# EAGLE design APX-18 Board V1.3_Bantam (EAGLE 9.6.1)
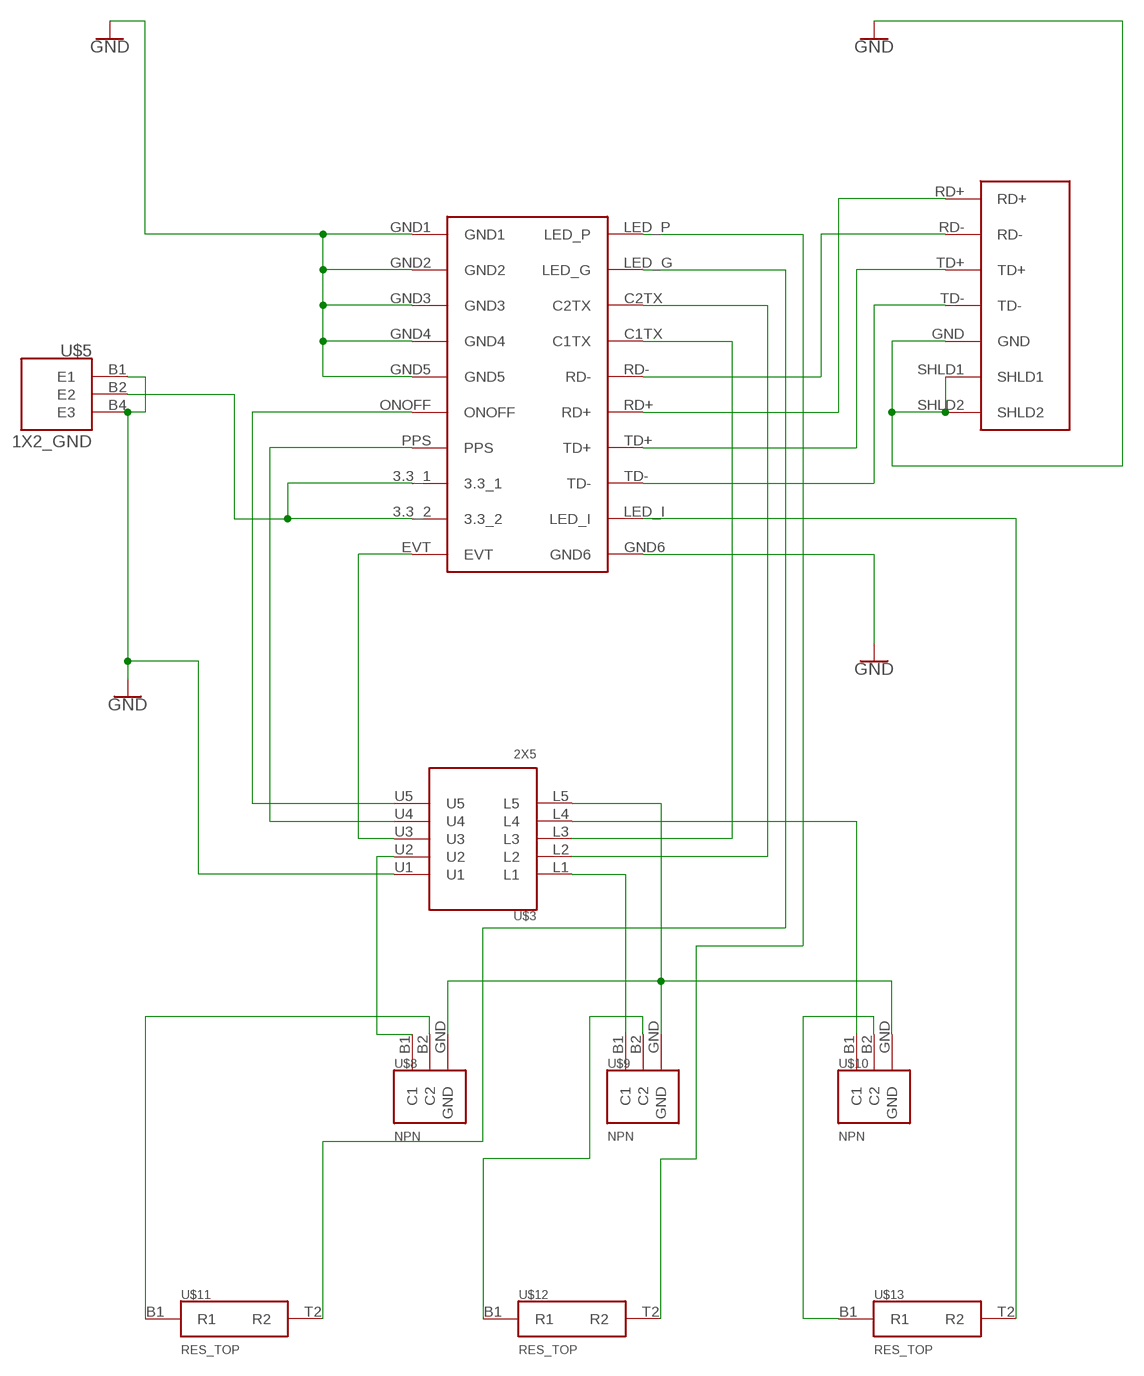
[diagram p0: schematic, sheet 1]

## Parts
U$1  APX18  [F_APX18]
U$2  MOLEX_MAG_ETH  [F_MOLEX_MAG_ETH]
U$3  2X5  [F_2X5]
U$5  1X2_GND  [F_1X2_GND]
U$8  NPN  [F_NPN]
U$9  NPN  [F_NPN]
U$10  NPN  [F_NPN]
U$11  RES_TOP  [F_RES]
U$12  RES_TOP  [F_RES]
U$13  RES_TOP  [F_RES]

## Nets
GND: U$1.GND1 U$1.GND2 U$1.GND3 U$1.GND4 U$1.GND5 U$1.GND6 U$2.GND U$2.SHLD1 U$2.SHLD2 U$3.U1 U$5.B1(E1) U$5.B4(E3)
N$1: U$1.TD- U$2.TD-
N$2: U$1.TD+ U$2.TD+
N$3: U$1.RD+ U$2.RD+
N$4: U$1.RD- U$2.RD-
N$5: U$1.3.3_1 U$1.3.3_2 U$5.B2(E2)
N$6: U$1.EVT U$3.U3
N$7: U$3.U2 U$8.B1(C1)
N$8: U$1.PPS U$3.U4
N$9: U$1.ONOFF U$3.U5
N$10: U$1.LED_I U$13.T2(R2)
N$11: U$1.C1TX U$3.L3
N$12: U$8.B2(C2) U$11.B1(R1)
N$13: U$1.C2TX U$3.L2
N$14: U$1.LED_G U$11.T2(R2)
N$15: U$1.LED_P U$12.T2(R2)
N$16: U$3.L1 U$9.B1(C1)
N$17: U$9.B2(C2) U$12.B1(R1)
N$18: U$3.L4 U$10.B1(C1)
N$19: U$10.B2(C2) U$13.B1(R1)
N$20: U$3.L5 U$8.GND U$9.GND U$10.GND

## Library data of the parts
U$1 = OpenMMS_Bantam:APX18
U$2 = OpenMMS_Bantam:MOLEX_MAG_ETH
U$3 = OpenMMS_Bantam:2X5
U$5 = OpenMMS_Bantam:1X2_GND
U$8-U$10 = OpenMMS_Bantam:NPN
U$11-U$13 = OpenMMS_Bantam:RES_TOP

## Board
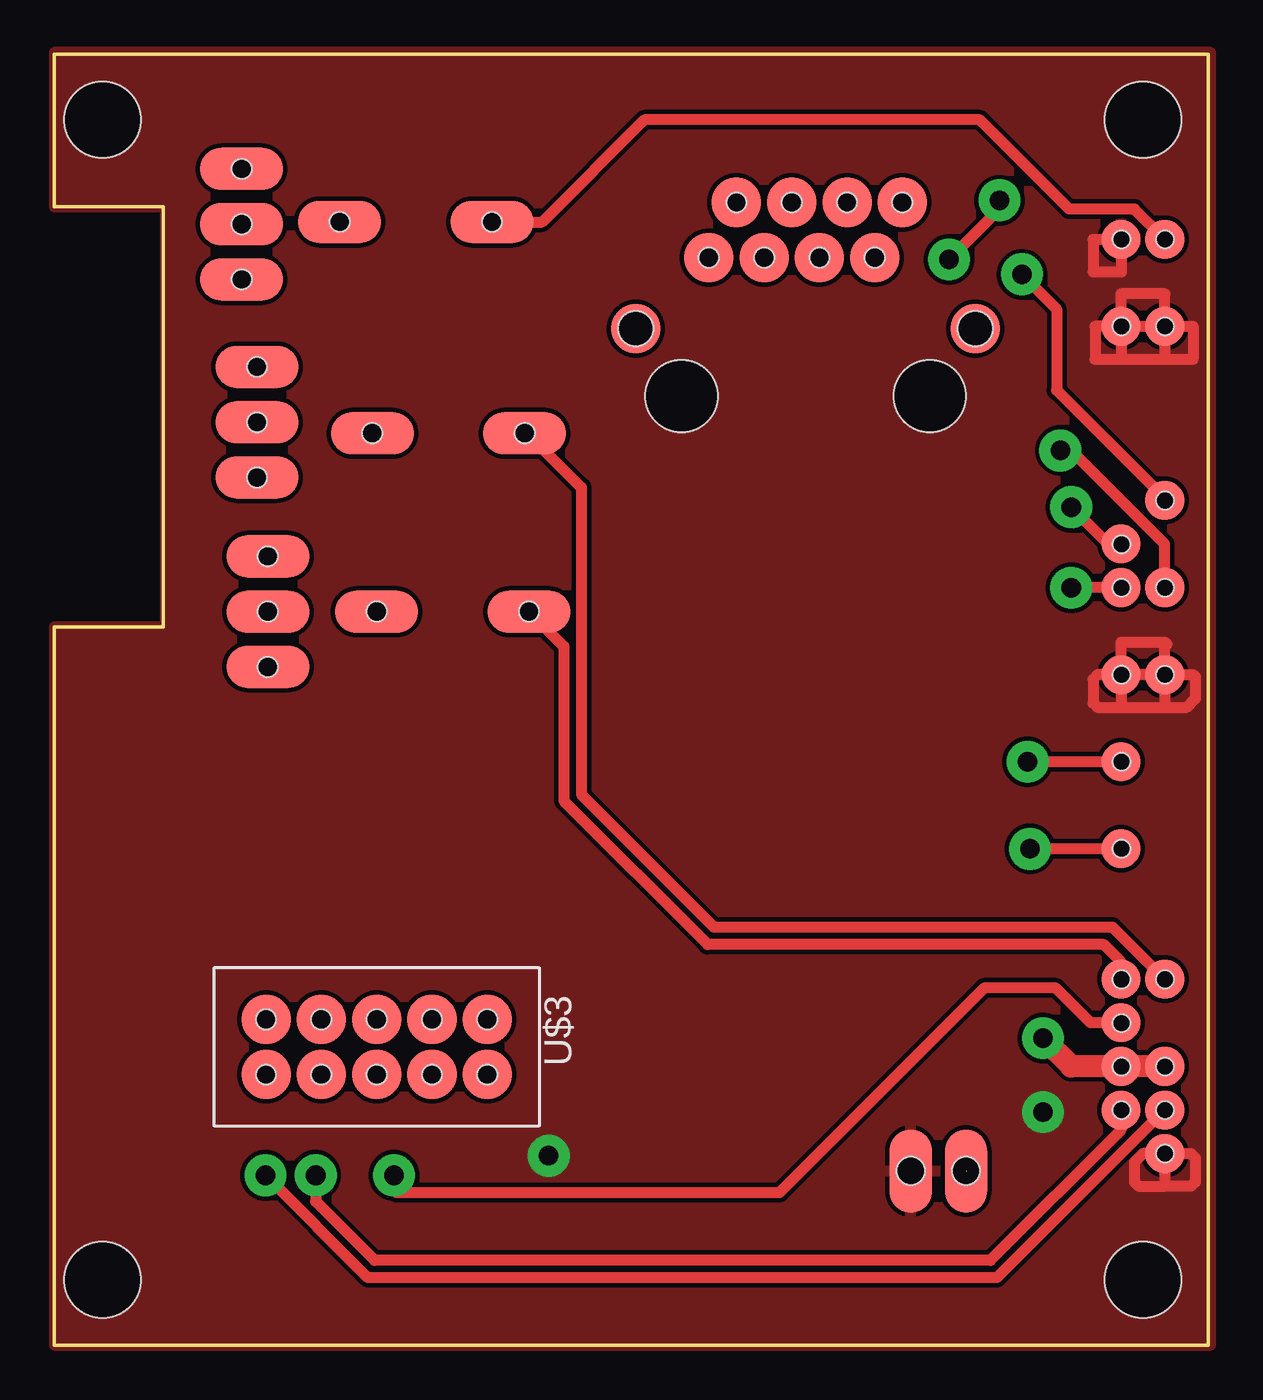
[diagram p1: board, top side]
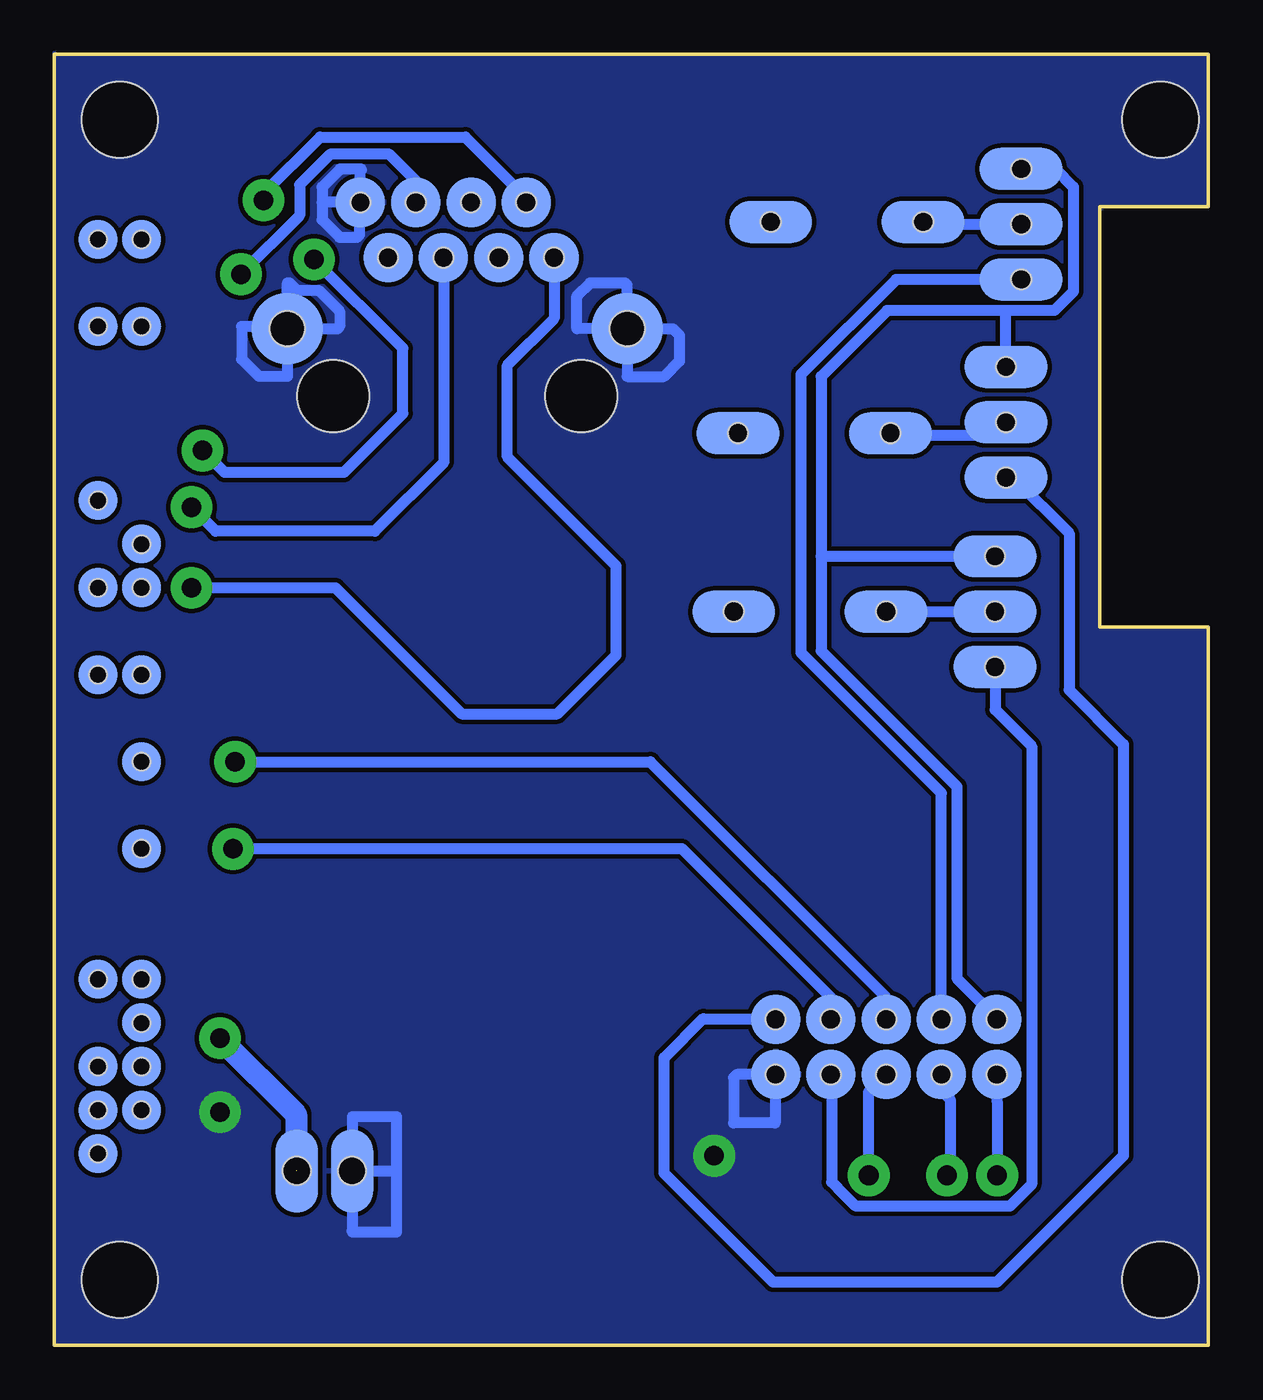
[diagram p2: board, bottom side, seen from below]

Size 53 x 59.3 mm. Coordinates in mm from the lower left corner, seen from the top.
Outline: 53,59.3 0,59.3 0,52.3 5,52.3 5,33 0,33 0,0 53,0 53,59.3
Copper layers (1*16): Top 0.035mm / dielectric 1.5mm / Bottom 0.035mm
Design rules "OpenMMS_Bantam": minimum track width 20mil, minimum drill 0.9mm, track to track 8mil, track to pad 8mil, pad to pad 8mil, via to via 8mil, smd to smd 8mil, copper to edge 0mil, drill to drill 0mil, minimum pad ring 20mil, minimum via ring 20mil, stop-mask expansion 4mil, vias tented up to drill 0mil, thermal gap 8mil
Holes 3.5 mm at 2.2,56.3 50,56.3 50,3 2.2,3

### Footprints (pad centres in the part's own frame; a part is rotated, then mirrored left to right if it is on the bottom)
F_APX18 = smd 1.8 x 1.8: 3.3_1 1.995,-37.995; 3.3_2 -0.005,-37.995; C1TX -0.005,-23.995; C2TX -0.005,-27.995; EVT -0.005,-35.995; GND1 1.995,-19.995; GND2 -0.005,-19.995; GND3 -0.005,0.005; GND4 -0.005,-3.995; GND5 1.995,-3.995; GND6 1.995,-41.995; LED_G -0.005,-33.995; LED_I 1.995,0.005; LED_P 1.995,-33.995; ONOFF 1.995,-39.995; PPS -0.005,-39.995; RD+ -0.005,-15.995; RD- 1.995,-15.995; TD+ -0.005,-13.995; TD- 1.995,-11.995 | smd 1.8 x 1.8 bottom: P$1 -0.005,-39.995; P$2 1.995,-39.995; P$3 -0.005,-37.995; P$4 1.995,-37.995; P$5 -0.005,-35.995; P$6 -0.005,-33.995; P$7 1.995,-33.995; P$8 -0.005,-27.995; P$9 -0.005,-23.995; P$11 -0.005,-19.995; P$12 1.995,-19.995; P$13 -0.005,-15.995; P$14 1.995,-15.995; P$15 -0.005,-13.995; P$16 1.995,-11.995; P$17 1.995,-3.995; P$18 -0.005,-3.995; P$19 1.995,0.005; P$20 -0.005,0.005; P$21 1.995,-41.995 | hole 0.8: 2,-42; 2,-40; 0,-40; 0,-38; 2,-38; 0,-36; 0,-34; 0,-28; 0,-24; 2,-20; 0,-20; 0,-16; 2,-16; 0,-14; 2,-12; 2,-4; 0,-4; 0,0; 2,0; 2,-34
F_MOLEX_MAG_ETH = smd 2.286 x 2.286 bottom: GND 4.445,0; P$11 -1.905,-2.54; P$12 -0.635,0; P$15 3.175,-2.54; RD+ -4.445,-2.54; RD- -3.175,0; TD+ 0.635,-2.54; TD- 1.905,0 | smd 2.286 x 2.286: P$1 -4.445,-2.54; P$2 -3.175,0; P$3 -1.905,-2.54; P$4 -0.635,0; P$5 0.635,-2.54; P$6 1.905,0; P$7 3.175,-2.54; P$8 4.445,0; P$9 7.8,-5.8; P$10 -7.8,-5.8 | smd 3.286 x 3.286 bottom: SHLD1 7.8,-5.8; SHLD2 -7.8,-5.8 | hole 0.9: -4.445,-2.54; -3.175,0; -1.905,-2.54; -0.635,0; 0.635,-2.54; 1.905,0; 3.175,-2.54; 4.445,0 | hole 3.3: -5.7,-8.9; 5.7,-8.9 | hole 1.6: -7.8,-5.8; 7.8,-5.8
F_2X5 = smd 2.286 x 2.286: B1 -5.08,-1.27; B2 -2.54,-1.27; B3 0,-1.27; B4 2.54,-1.27; B5 5.08,-1.27; B6 5.08,1.27; B7 2.54,1.27; B8 0,1.27; B9 -2.54,1.27; B20 -5.08,1.27 | smd 2.286 x 2.286 bottom: L1 -5.08,-1.27; L2 -2.54,-1.27; L3 0,-1.27; L4 2.54,-1.27; L5 5.08,-1.27; U1 -5.08,1.27; U2 -2.54,1.27; U3 0,1.27; U4 2.54,1.27; U5 5.08,1.27 | hole 0.9: -5.08,-1.27; -2.54,-1.27; 0,-1.27; 2.54,-1.27; 5.08,-1.27; 5.08,1.27; 2.54,1.27; 0,1.27; -2.54,1.27; -5.08,1.27
F_1X2_GND = smd 3.81 x 1.93 bottom: B1 0,1.27; B2 0,-1.27 | smd 3.81 x 1.93: B4 0,1.27; B5 0,-1.27 | hole 1.27: 0,1.27; 0,-1.27
F_NPN = smd 1.93 x 3.81 bottom: B1 -2.54,0; B2 0,0; GND 2.54,0 | smd 1.93 x 3.81: B4 -2.54,0; B5 0,0; B6 2.54,0 | hole 0.9: -2.54,0; 0,0; 2.54,0
F_RES = smd 1.93 x 3.81 bottom: B1 0,3.5; B2 0,-3.5 | smd 1.93 x 3.81: T1 0,3.5; T2 0,-3.5 | hole 0.9: 0,3.5; 0,-3.5

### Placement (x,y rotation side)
U$1  49,50.8 0 top
U$2  34.5,52.5 0 top
U$3  14.8,13.7 180 top
U$5  40.6,8 90 top
U$8  9.8,33.7 90 top
U$9  9.3,42.4 90 top
U$10  8.6,51.5 90 top
U$11  18.3,33.7 90 top
U$12  18.1,41.9 90 top
U$13  16.6,51.6 90 top

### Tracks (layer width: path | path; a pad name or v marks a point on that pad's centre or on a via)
GND  (via drill 0.9)
  Top 0.508: U$1.GND6 52.2,8.8 52.4,8.6 52.4,7.5 52.2,7.3 51,7.3 | 51,7.3 50.99,7.3 | U$1.GND6 50.01,8.8 49.6,8.4 49.6,7.5 49.8,7.3 51,7.3 | U$1.GND6 51,7.3 | U$1.GND2 | U$1.GND2 47.9,30.8 47.7,30.6 47.7,29.5 47.9,29.3 49,29.3 | 49,29.3 51,29.3 | 51,29.3 52,29.3 52.4,29.7 52.4,30.7 52.3,30.8 U$1.GND1 | U$1.GND1 U$1.GND2 | U$1.GND2 48.99,29.3 49,29.3 | U$1.GND1 50.99,29.3 51,29.3 | U$1.GND2 48.99,32.3 49,32.3 51,32.3 | 51,32.3 51.1,32.2 | U$1.GND1 51,32.3 | U$1.GND4 47.8,46.8 47.8,45.3 48.9,45.3 | 48.9,45.3 51,45.3 | 51,45.3 52.3,45.3 52.3,46.8 U$1.GND5 | U$1.GND5 50.99,45.3 51,45.3 | U$1.GND4 48.99,45.4 48.9,45.3 | U$1.GND4 48.99,48.3 49,48.3 51,48.3 U$1.GND5 | U$1.GND4 U$1.GND5 | U$1.GND3 47.7,50.8 47.7,49.3 49,49.3 48.99,49.3 U$1.GND3
  Bottom 0.508: U$5.B1 39.3,8.03 39.3,10.5 37.3,10.5 37.3,7.9 | 37.3,7.9 37.3,5.2 39.3,5.2 39.33,5.23 U$5.B1 | U$5.B1 37.4,8 37.3,7.9 | U$2.GND 38.95,53.95 38.9,54 38.93,54.03 39.87,54.03 40.7,53.2 40.7,52.5 | U$2.GND 40.7,52.5 | 40.7,52.5 40.7,51.7 39.9,50.9 39.1,50.9 39,51 39,52.45 U$2.GND | U$2.SHLD2 26.7,48.7 26.8,48.8 28.4,48.8 29,48.2 29,46.7 U$2.SHLD2 | U$2.SHLD2 24.6,46.7 24.3,46.4 24.3,45.2 25,44.5 26.7,44.5 U$2.SHLD2 | U$2.SHLD1 42.3,48.8 42.2,48.8 41.87,48.47 40.87,48.47 39.9,47.5 39.9,46.8 40,46.7 U$2.SHLD1 | U$2.SHLD1 42.4,46.8 44.4,46.8 44.4,45.3 43.6,44.5 42.3,44.5 U$2.SHLD1 | U$3.U1 21.67,12.43 21.8,12.3 21.8,10.2 19.9,10.2 19.9,12.41 U$3.U1
  other vias: 45.4,10.7 22.7,8.7
  pour Bottom: 52.9,59.3 53,59.4 53,0.1 52.9,0 0.1,0 0,0.1 0,32.9 0.1,33 5.1,33 5.1,52 4.8,52.3 0,52.3 0,59.2 0.1,59.3
  pour Top: 0,59.4 0,52.3 5.1,52.3 5.1,33 0,33 0,0 53.1,0 53.1,59.4
N$1  (via drill 0.9)
  Top 0.508: v44.43,49.2 46.03,47.6 46.03,43.87 50.99,38.91 U$1.TD-
  Bottom 0.508: v44.43,49.2 41.73,51.9 41.73,53.3 40.3,54.74 37.65,54.74 36.41,53.5 U$2.TD-
N$2  (via drill 0.9)
  Top 0.508: v46.7,38.5 48.4,36.8 U$1.TD+
  Bottom 0.508: v46.7,38.5 45.6,37.4 38.28,37.4 35.1,40.58 35.1,49 35.13,49.03 U$2.TD+
N$3  (via drill 0.9)
  Top 0.508: v46.7,34.8 U$1.RD+
  Bottom 0.508: U$2.RD+ 30.05,47.16 32.2,45.02 32.2,40.8 27.2,35.8 27.2,31.7 29.9,29 34.3,29 40.1,34.8 v46.7,34.8
N$4  (via drill 0.9)
  Top 0.508: v43.4,52.6 43.4,52.2 v41.08,49.88 | U$1.RD- 50.99,36.8 46.7,41.1 v46.2,41.1
  Bottom 0.508: v43.4,52.6 43.4,52.9 40.8,55.5 34.13,55.5 31.32,52.7 U$2.RD- | v46.2,41.1 45.2,40.1 39.7,40.1 37,42.8 37,45.8 v41.08,49.88
N$5  (via drill 0.9)  (1 unrouted)
  Top 1: v45.4,14.1 46.7,12.8 U$1.3.3_2 U$1.3.3_1
  Bottom 1: v45.4,14.1 41.9,10.6 41.9,8
N$6  (via drill 0.9)
  Top 0.508: v15.6,7.8 15.6,7.1 15.7,7 33.3,7 42.7,16.4 46,16.4 47.59,14.8 U$1.EVT
  Bottom 0.508: v15.6,7.8 15.6,11.63 15.5,11.73 U$3.U3
N$7
  Bottom 0.508: U$8.B1 9.8,29.2 8.12,27.52 8.12,7.38 9.11,6.38 16.19,6.38 17.02,7.21 17.3,7.5 17.3,12.39 U$3.U2
N$8  (via drill 0.9)
  Top 0.508: U$1.PPS 48.99,9.89 42.99,3.89 14.71,3.89 12,6.6 v12,7.8
  Bottom 0.508: v12,7.8 11.86,7.94 11.86,11.3 12.26,11.7 U$3.U4
N$9  (via drill 0.9)
  Top 0.508: v9.7,7.8 14.4,3.1 43.29,3.1 U$1.ONOFF
  Bottom 0.508: v9.7,7.8 9.7,11.2 9.72,11.22 U$3.U5
N$10
  Top 0.508: U$1.LED_I 49.6,52.2 46.6,52.2 42.5,56.3 27.1,56.3 22.4,51.6 U$13.T2
N$11  (via drill 0.9)
  Top 0.508: U$1.C1TX v44.7,26.8
  Bottom 0.508: v44.7,26.8 25.63,26.8 14.87,16.03 14.8,15.97 U$3.L3
N$12
  Bottom 0.508: U$11.B1 U$8.B2
N$13  (via drill 0.9)
  Top 0.508: U$1.C2TX v44.8,22.8
  Bottom 0.508: v44.8,22.8 24.17,22.8 17.34,15.97 U$3.L2
N$14
  Top 0.508: U$11.T2 23.4,32.1 23.4,25 30,18.4 48.2,18.4 48.99,17.61 U$1.LED_G
N$15
  Top 0.508: U$1.LED_P 48.6,19.2 30.3,19.2 24.2,25.3 24.2,39.4 21.7,41.9 U$12.T2
N$16
  Bottom 0.508: U$9.B1 8.96,39.86 6.4,37.3 6.4,30.1 3.9,27.6 3.9,8.7 9.71,2.89 19.99,2.89 25,7.9 25,13.2 23.2,15 23.17,14.97 U$3.L1
N$17
  Bottom 0.508: U$9.B2 9.9,41.8 14.5,41.8 U$12.B1
N$18
  Bottom 0.508: U$10.B1 14.34,48.96 18.7,44.6 18.7,31.8 12.26,25.36 U$3.L4
N$19
  Bottom 0.508: U$13.B1 13,51.5 U$10.B2
N$20
  Bottom 0.508: U$10.GND 7.04,54.04 6.2,53.2 6.2,48.41 7.07,47.54 9.3,47.54 | 9.3,47.54 14.76,47.54 17.79,44.51 17.79,36.24 | 17.79,36.24 17.79,31.89 11.55,25.66 11.55,16.85 10.5,15.8 9.72,15.02 U$3.L5 | U$9.GND 9.3,47.54 | U$8.GND 17.79,36.24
